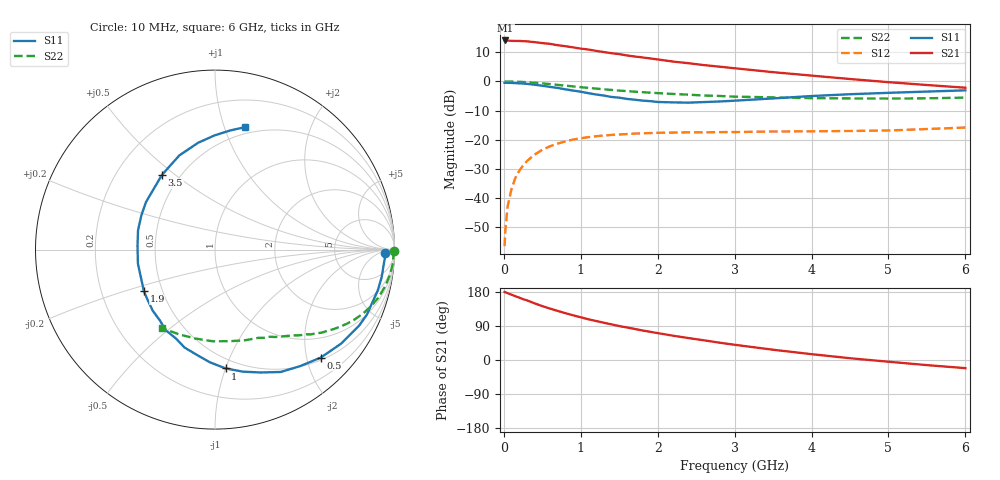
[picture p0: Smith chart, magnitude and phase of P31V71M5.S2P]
! SIEMENS Small Signal Semiconductors
! BFP181
! Si NPN RF Bipolar Junction Transistor in SOT143
! VCE = 1.75 V  IC = 1.5 mA
! Common Emitter S-Parameters:  March  1996
# GHz  S  MA  R  50
!  f  S11  S21  S12  S22
! GHz  MAG  ANG  MAG  ANG  MAG  ANG  MAG  ANG
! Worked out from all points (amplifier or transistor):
!   36 points, 10 MHz to 6 GHz, reference 50 ohm
!   highest |S21| = 14.0 dB at 20 MHz (marker M1)
!   |S21| within 3 dB of that: start of sweep to 1.063 GHz
!   unconditionally stable (mu >= 1): 2.615 GHz to end of sweep
!   at 250 MHz: K = 0.11, MSG = 21.3 dB, |S12| = -28.8 dB
!   at 1.4 GHz: K = 0.59, MSG = 14.0 dB, |S12| = -18.3 dB
!   at 6 GHz: K = 1.20, MAG = 4.1 dB, |S12| = -15.8 dB
!   S11 on the Smith chart (normalised r, x): 10 MHz: 31, -12; 500 MHz: 0.55, -2.27; 1 GHz: 0.42, -1.00; 1.9 GHz: 0.39, -0.23; 3.5 GHz: 0.40, +0.45; 6 GHz: 0.44, +1.18
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0.01  0.945 -1.2  5.008 179.4  0.0015 87.7  0.9969 -0.4
0.02  0.9497 -2.0  5.03 179.0  0.0029 81.9  0.9954 -0.9
0.05  0.9445 -4.4  5.007 176.1  0.0073 88.7  0.9943 -2.1
0.1  0.9413 -9.3  4.953 172.3  0.0143 84.3  0.9941 -4.3
0.15  0.9349 -14.2  4.936 168.4  0.0222 81.0  0.9888 -6.4
0.25  0.9206 -23.2  4.89 160.6  0.0362 75.3  0.9758 -10.6
0.3  0.9078 -27.8  4.855 157.4  0.0431 72.7  0.9674 -12.6
0.4  0.877 -36.6  4.709 149.4  0.0556 67.6  0.9487 -16.4
0.5  0.8421 -45.6  4.533 142.2  0.0672 61.9  0.9244 -20.0
0.6  0.8043 -53.8  4.403 135.7  0.0773 57.3  0.8988 -23.3
0.8  0.73 -69.7  4.012 123.6  0.0935 48.8  0.8454 -29.1
1  0.6645 -84.9  3.643 112.7  0.1059 41.5  0.7962 -33.8
1.1  0.6281 -92.7  3.513 107.4  0.1109 38.6  0.7733 -35.8
1.3  0.5716 -107.2  3.182 98.3  0.118 33.1  0.7316 -39.6
1.5  0.5262 -121.5  2.931 89.6  0.1231 28.9  0.695 -42.8
1.9  0.4591 -149.7  2.478 74.5  0.1302 21.8  0.6405 -48.5
2.2  0.4366 -169.7  2.187 64.1  0.1326 18.1  0.6093 -52.6
2.8  0.4525 155.0  1.789 45.8  0.1352 12.9  0.5629 -60.8
3.5  0.5108 125.3  1.439 27.1  0.1384 9.4  0.5319 -71.8
4.5  0.6029 98.9  1.099 4.7  0.1413 6.3  0.5109 -91.5
5.5  0.6693 82.7  0.867 -13.5  0.1526 6.9  0.5133 -113.2
6  0.7022 76.3  0.779 -21.5  0.1618 5.7  0.5272 -124.3
